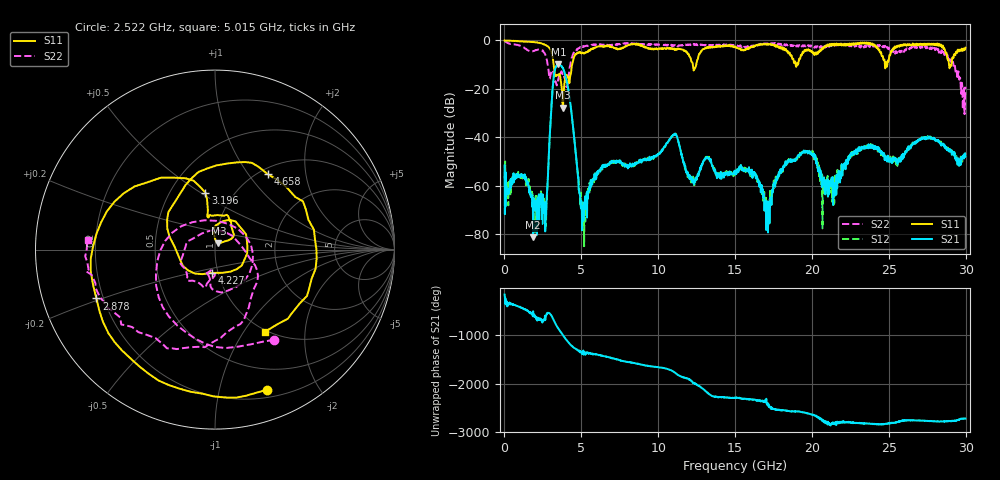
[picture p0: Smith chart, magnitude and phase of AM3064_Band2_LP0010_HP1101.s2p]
# Hz S DB R 50.0
!freq dBS11 angS11 dBS21 angS21 dBS12 angS12 dBS22 angS22
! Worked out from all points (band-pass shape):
!   1600 points, 10 MHz to 29.98 GHz, reference 50 ohm
!   highest |S21| = -9.83 dB at 3.515 GHz (marker M1); lowest = -81.4 dB at 1.866 GHz (marker M2)
!   |S21| within 3 dB of the highest: 3.26 GHz to 3.884 GHz (624.1 MHz wide, 17.5 % of centre)
!   lowest |S11| = -27.9 dB at 3.796 GHz (marker M3), VSWR 1.08, Z = 51.8 + j3.7 ohm
!   |S11| at or under -10 dB: 3.199 GHz to 4.398 GHz (1.2 GHz wide, 31.6 % of centre); 12.25 GHz to 12.47 GHz (224.1 MHz wide, 1.81 % of centre); 28.91 GHz to 29.08 GHz (166.4 MHz wide, 0.574 % of centre)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
!   |S22| runs from -30.5 to -0.2 dB; largest |S21 - S12| = 0.012
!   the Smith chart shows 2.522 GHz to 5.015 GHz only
!   S11 on the Smith chart (normalised r, x): 2.522 GHz: 0.27, -1.40; 2.878 GHz: 0.17, -0.19; 3.196 GHz: 0.74, +0.52; 4.227 GHz: 0.94, -0.25; 4.658 GHz: 1.09, +1.24; 5.015 GHz: 0.98, -1.26
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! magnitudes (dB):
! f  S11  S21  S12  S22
! 10 MHz  0.0  -51.7  -57.2  -0.2
! 1.866 GHz  -0.7  -81.4  -71.8  -4.4
! 2.522 GHz  -1.6  -69.5  -66.4  -4.4
! 2.878 GHz  -2.9  -48.5  -48.3  -12.8
! 3.196 GHz  -9.9  -15.7  -15.4  -13.7
! 3.515 GHz  -14.3  -9.8  -10.1  -15.7
! 3.796 GHz  -27.9  -11.5  -11.4  -13.8
! 4.227 GHz  -17.7  -23.5  -23.4  -11.6
! 4.658 GHz  -5.8  -48.1  -48.0  -4.3
! 5.015 GHz  -5.4  -69.0  -66.8  -3.0
! 6.402 GHz  -2.5  -52.1  -51.7  -1.8
! 10 GHz  -3.5  -47.0  -47.1  -1.8
! 11.09 GHz  -4.0  -38.6  -38.6  -1.9
! 15 GHz  -2.6  -55.0  -55.4  -1.9
! 17.12 GHz  -1.6  -66.6  -75.2  -1.3
! 18.27 GHz  -4.1  -51.6  -51.4  -2.1
! 19.99 GHz  -4.4  -46.8  -46.9  -2.2
! 21.3 GHz  -1.9  -58.7  -58.3  -1.6
! 22.9 GHz  -1.6  -45.3  -46.0  -2.4
! 25 GHz  -8.1  -50.0  -48.8  -2.9
! 28.56 GHz  -3.0  -42.9  -43.2  -4.8
! 29.98 GHz  -3.1  -47.8  -47.8  -19.2
